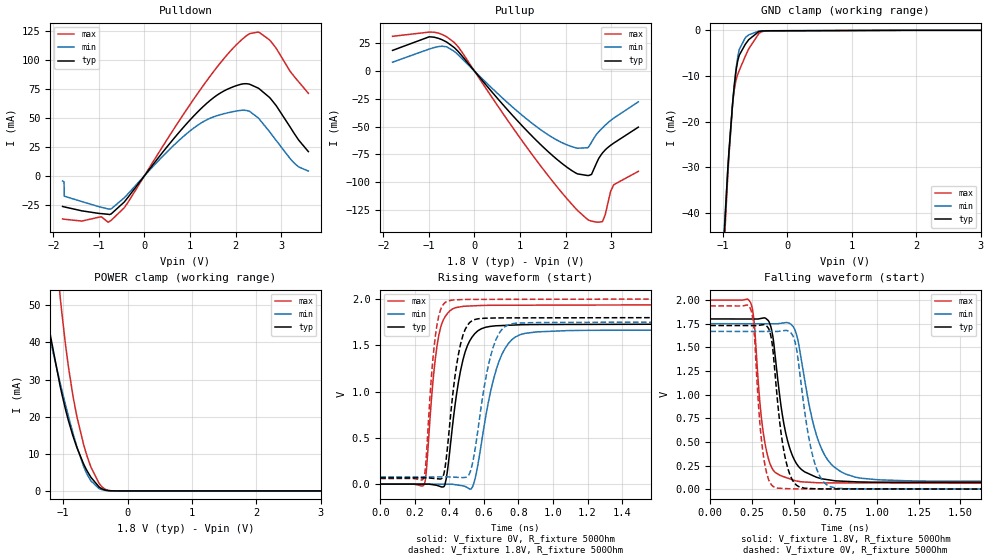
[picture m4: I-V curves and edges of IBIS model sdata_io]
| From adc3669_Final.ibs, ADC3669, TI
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|   sdata_io Model
[Model]   sdata_io
Model_type   I/O
Polarity   Non-Inverting
Enable   Active-High
Vinl = 0.4
Vinh = 1.3
Vmeas = 0.9
Vref = 0
Cref = 2pF
Rref = 100000
|   typ   min   max
C_comp   0.36952pF   0.32036pF   0.438168pF
| Where C_comp = 0.36952pF at 1.8V, 27C and nominal process
| Where C_comp = 0.438168pF at 1.75V, 105C and weak process
| Where C_comp = 0.32036pF at 2V, -40C and strong process
[Voltage Range]   1.8   1.75   2
|Junction Temperature
[Temperature Range]   27   105   -40
[Pullup Reference]   1.8   1.75   2
[Pulldown Reference]   0   0   0
[Power Clamp Reference]   1.8   1.75   2
[GND Clamp Reference]   0   0   0
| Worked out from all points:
|   slope of the pulldown table from 0 to 0.27 V, typ, clamps not added: 19.6 ohm
|   slope of the pullup table from 0 to 0.27 V, typ, clamps not added: 20.3 ohm
|   GND clamp passes 1 mA (typ) near -0.51 V on its own axis
|   POWER clamp passes 1 mA (typ) near -0.44 V on its own axis
|   falling waveform, V_fixture 1.8V, R_fixture 500Ohm: 20-80 % time 93.7ps typ, 129ps min, 62.1ps max; typ from 1.8 V to 0.067 V
|   rising waveform, V_fixture 0V, R_fixture 500Ohm: 20-80 % time 83.2ps typ, 113ps min, 57.3ps max; typ from 0 V to 1.73 V
|   rising waveform, V_fixture 1.8V, R_fixture 500Ohm: 20-80 % time 68.2ps typ, 91.9ps min, 48.2ps max; typ from 0.067 V to 1.8 V
|   falling waveform, V_fixture 0V, R_fixture 500Ohm: 20-80 % time 67.5ps typ, 87.9ps min, 48.7ps max; typ from 1.73 V to 0 V
[Pulldown]
|   Voltage   I(typ)   I(min)   I(max)
-1.8V     -26.42mA   -4.429mA   -37.12mA
-1.768V   -26.76mA   -5.122mA   -37.38mA
-1.762V   -26.81mA   -17.57mA   -37.42mA
-995.4mV  -32.47mA   -26.68mA   -35.63mA
-801mV    -33.16mA   -28.52mA   -39.98mA
-444.6mV  -22.59mA   -18.97mA   -27.55mA
1.143V    54.01mA    42.86mA    69.53mA
1.748V    73.14mA    53.49mA    101.1mA
2.309V    78.89mA    55.52mA    122.5mA
2.752V    67.22mA    37.73mA    116.8mA
3.292V    36.27mA    10.82mA    85.38mA
3.6V      20.84mA    4.071mA    71.05mA
[GND Clamp]
|   Voltage   I(typ)   I(min)   I(max)
-1.8V     -307.5mA   -284.6mA   -324.4mA
-1.049V   -62.24mA   -59.12mA   -65.62mA
-930.6mV  -31.18mA   -31.17mA   -32.62mA
-909mV    -26.44mA   -26.63mA   -27.43mA
-855mV    -16.4mA    -16.42mA   -16.62mA
-828mV    -12.31mA   -12.16mA   -13.09mA
-795.6mV  -8.491mA   -8.026mA   -10.68mA
-747mV    -5.385mA   -4.114mA   -8.697mA
-601.2mV  -2.026mA   -988.8uA   -4.018mA
-444.6mV  -271uA     -166.9uA   -696uA
-336.6mV  -112.4uA   -94.4uA    -160.7uA
3.6V      0A         0A         0A
[Pullup]
|   Voltage   I(typ)   I(min)   I(max)
-1.8V     18.65mA    7.994mA    31.34mA
-995.4mV  30.88mA    19.86mA    35.13mA
-714.6mV  28.28mA    22.41mA    33.06mA
-444.6mV  21.2mA     17.84mA    25.8mA
1.445V    -65.92mA   -52.56mA   -85mA
2.126V    -89.3mA    -67.88mA   -119.4mA
2.488V    -94.11mA   -69.07mA   -133.8mA
2.574V    -92.85mA   -63.87mA   -135.2mA
2.812V    -73.8mA    -51.25mA   -135.4mA
2.99V     -66.9mA    -44.54mA   -108.5mA
3.06V     -64.86mA   -42.34mA   -102.4mA
3.6V      -50.5mA    -27.7mA    -90.34mA
[POWER Clamp]
|   Voltage   I(typ)   I(min)   I(max)
-1.8V     138.2mA    94.51mA    232.4mA
-1.352V   59.33mA    52.61mA    115.6mA
-1.206V   42.72mA    41.06mA    82.91mA
-1.049V   28.47mA    29.29mA    52.83mA
-919.8mV  19.06mA    20.22mA    33.65mA
-849.6mV  14.91mA    15.69mA    25.78mA
-784.8mV  11.61mA    11.83mA    19.89mA
-622.8mV  5.232mA    4.295mA    9.064mA
-444.6mV  1.123mA    677.4uA    2.128mA
-347.4mV  235.5uA    146.2uA    478.2uA
-217.8mV  19.22uA    19.59uA    28.19uA
3.6V      0A         0A         0A
[Ramp]
R_load = 500
|   typ   min   max
dV/dt_r   1.03825/8.31499e-11   1.00101/1.12759e-10   1.16272/5.72861e-11
dV/dt_f   1.03972/9.36056e-11   1.00335/1.29143e-10   1.16357/6.20742e-11
[Falling Waveform]
V_fixture = 1.8V
V_fixture_min = 1.75V
V_fixture_max = 2V
R_fixture = 500Ohm
C_fixture = 0F
|   Time   V(typ)   V(min)   V(max)
0s        1.8V       1.75V      2V
244.8ps   1.799V     1.749V     1.961V
311.1ps   1.808V     1.749V     686.4mV
351.7ps   1.772V     1.749V     304.2mV
442.2ps   682.3mV    1.759V     130.5mV
497.6ps   335.6mV    1.719V     96.56mV
639.4ps   124.7mV    557.6mV    68.29mV
810.4ps   82.82mV    160.3mV    65.77mV
1.292ns   72.88mV    85.49mV    64.15mV
50ns      67.13mV    77.73mV    60.7mV
[Rising Waveform]
V_fixture = 0V
V_fixture_min = 0V
V_fixture_max = 0V
R_fixture = 500Ohm
C_fixture = 0F
|   Time   V(typ)   V(min)   V(max)
0s        100.2nV    320.8nV    1.381uV
254.3ps   214uV      -270uV     -3.17mV
319ps     -10.28mV   -338.9uV   1.358V
368.2ps   -28mV      -391.2uV   1.785V
478.7ps   1.343V     -18.56mV   1.921V
537.3ps   1.603V     -15.15mV   1.927V
589.5ps   1.682V     488.8mV    1.931V
760.7ps   1.718V     1.559V     1.933V
1.175ns   1.726V     1.662V     1.935V
50ns      1.73V      1.668V     1.938V
[Rising Waveform]
V_fixture = 1.8V
V_fixture_min = 1.75V
V_fixture_max = 2V
R_fixture = 500Ohm
C_fixture = 0F
|   Time   V(typ)   V(min)   V(max)
0s        67.13mV    77.73mV    60.7mV
251.4ps   67.53mV    78.03mV    64.8mV
311.1ps   61.33mV    78.11mV    1.473V
361.5ps   73.13mV    78.17mV    1.931V
432.9ps   1.17V      74.61mV    1.991V
482.1ps   1.626V     70.57mV    1.995V
532.5ps   1.767V     213.9mV    1.996V
670.5ps   1.796V     1.565V     1.997V
868.5ps   1.797V     1.745V     1.998V
50ns      1.8V       1.75V      2V
[Falling Waveform]
|Gnd
V_fixture = 0V
V_fixture_min = 0V
V_fixture_max = 0V
R_fixture = 500Ohm
C_fixture = 0F
|   Time   V(typ)   V(min)   V(max)
0s        1.73V      1.668V     1.938V
244.8ps   1.73V      1.668V     1.891V
263.6ps   1.73V      1.668V     1.653V
304.3ps   1.736V     1.668V     564.4mV
351.7ps   1.691V     1.668V     93.54mV
432.9ps   490.7mV    1.674V     7.988mV
482.1ps   134.5mV    1.655V     3.587mV
636.5ps   3.574mV    220mV      2.334mV
837.9ps   2.493mV    3.089mV    2.003mV
50ns      100.2nV    320.8nV    1.381uV
